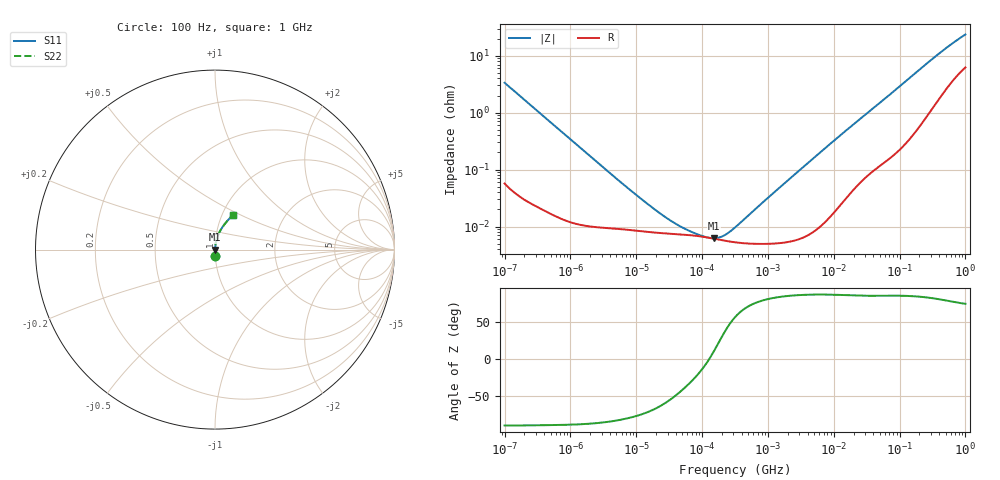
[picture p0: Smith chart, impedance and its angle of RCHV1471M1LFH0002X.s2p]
! RCHV1471M1LFH0002X  S-PARAMETER MODEL  (AEC-Q200 qualified)
! Model Generated by ELNA Corporation (http://www.ty-top.com)
! Version 1.0
! ELNA Control No. 240229
! Copyright (c) 2024 ELNA CO.,LTD. All Rights Reserved.
! Products Name : CONDUCTIVE POLYMER HYBRID ALUMINUM ELECTROLYTIC CAPACITORS
! Characteristics :
!  Capacitance  :  470uF  ,  Rated voltage  :  10V
!  Operating Temp. Range  :  -55 to +105 degC  ,  Endurance  :  5000hr at 105 degC
!  Dimension D  :  10mm  ,  Dimension L  :  10mm
! Frequency Range : 100Hz - 1GHz
! External Node Assignments :
!  1  o---| |---o  2
# MHz S RI R 50
!Freq[MHz].  S11 Real  S11 Imag  S21 Real  S21 Imag  S12 Real  S12 Imag  S22 Real  S22 Imag
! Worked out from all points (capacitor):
!   401 points, 100 Hz to 1 GHz, reference 50 ohm
!   read as one part in series: C = 475 uF near 108 Hz
!   lowest |Z| = 6.25 mohm at 153.1 kHz (marker M1)
!   series resonance near 127.7 kHz, so ESL is about 3.3 nH
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0.0001  0.00169 -0.0334  0.9983 0.0334  0.9983 0.0334  0.00169 -0.0334
0.000113  0.00137 -0.0296  0.9986 0.0296  0.9986 0.0296  0.00137 -0.0296
0.000309  0.000341 -0.0109  0.9997 0.0109  0.9997 0.0109  0.000341 -0.0109
0.001488  0.000111 -0.00229  0.9999 0.00229  0.9999 0.00229  0.000111 -0.00229
0.007161  8.85e-05 -0.000484  0.9999 0.000484  0.9999 0.000484  8.85e-05 -0.000484
0.013646  8.16e-05 -0.000257  0.9999 0.000257  0.9999 0.000257  8.16e-05 -0.000257
0.022131  7.74e-05 -0.000158  0.9999 0.000158  0.9999 0.000158  7.74e-05 -0.000158
0.035892  7.45e-05 -9.45e-05  0.9999 9.45e-05  0.9999 9.45e-05  7.45e-05 -9.45e-05
0.043904  7.34e-05 -7.49e-05  0.9999 7.49e-05  0.9999 7.49e-05  7.34e-05 -7.49e-05
0.047588  7.29e-05 -6.78e-05  0.9999 6.78e-05  0.9999 6.78e-05  7.29e-05 -6.78e-05
0.153109  6.12e-05 1.27e-05  0.9999 -1.27e-05  0.9999 -1.27e-05  6.12e-05 1.27e-05
0.316228  5.3e-05 8.05e-05  0.9999 -8.05e-05  0.9999 -8.05e-05  5.3e-05 8.05e-05
0.356862  5.21e-05 9.57e-05  0.9999 -9.57e-05  0.9999 -9.57e-05  5.21e-05 9.57e-05
1.017419  4.99e-05 0.000322  1 -0.000322  1 -0.000322  4.99e-05 0.000322
4.704354  8.02e-05 0.00152  0.9999 -0.00152  0.9999 -0.00152  8.02e-05 0.00152
15.13561  0.000328 0.00477  0.9997 -0.00477  0.9997 -0.00477  0.000328 0.00477
69.9842  0.00196 0.0203  0.998 -0.0203  0.998 -0.0203  0.00196 0.0203
176.8072  0.00713 0.0496  0.9929 -0.0496  0.9929 -0.0496  0.00713 0.0496
395.8221  0.0277 0.1025  0.9723 -0.1025  0.9723 -0.1025  0.0277 0.1025
668.3439  0.0612 0.1514  0.9388 -0.1514  0.9388 -0.1514  0.0612 0.1514
922.5714  0.0913 0.1843  0.9087 -0.1843  0.9087 -0.1843  0.0913 0.1843
1000  0.0998 0.1928  0.9002 -0.1928  0.9002 -0.1928  0.0998 0.1928
